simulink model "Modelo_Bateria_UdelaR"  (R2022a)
settings: Solver=VariableStepAuto  StartTime=0.0  StopTime=inf  RelTol=1e-3
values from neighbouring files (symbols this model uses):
  a = x(1)    [Cycling_LiFePO4.m]    (also in Parametros_A123.m = 2.09162011618e-08; Parametros_A123_pack.m = 2.09162011618e-08)
  A = @(x) x(1)    [Cycling_LiFePO4.m]    (also in LMFsolve.m = J'*J; Parametros_A123.m = 0.3446; Parametros_A123_pack.m = 0.3446)
  Alpha = 1093.6    [Parametros_A123.m]    (also in Parametros_A123_pack.m)
  b = x(2)    [Cycling_LiFePO4.m]    (also in Parametros_A123.m = -1.21794950859e-05; Parametros_A123_pack.m = -1.21794950859e-05)
  B = @(x) x(2)    [Cycling_LiFePO4.m]    (also in Parametros_A123.m = 13.0435; Parametros_A123_pack.m = 13.0435)
  Beta = 8390.6    [Parametros_A123.m]    (also in Parametros_A123_pack.m)
  c = x(3)    [Cycling_LiFePO4.m]    (also in Parametros_A123.m = 0.00180276688394; Parametros_A123_pack.m = 0.00180276688394)
  d = x(4)    [Cycling_LiFePO4.m]    (also in LMFsolve.m = (A+l*D)\v; Parametros_A123.m = -1.70817769928e-06; Parametros_A123_pack.m = -1.70817769928e-06)
  dE_dT = 0.000010001    (= 1.0001e-05)    [Parametros_A123.m]    (also in Parametros_A123_pack.m)
  dQ_dT = 0.0037    [Parametros_A123.m]    (also in Parametros_A123_pack.m)
  Eo = 3.3678    [Parametros_A123.m]    (also in Parametros_A123_pack.m)
  f = x(1)*Q0    [Calendar_LiFePO4.m]    (also in Cycling_LiFePO4.m = f*(exp(g)-1)/(g*exp(0.5)); LMFsolve.m = '; Parametros_A123.m = 5980801.16971; Parametros_A123_pack.m = 5980801.16971)
  g = x(2)    [Calendar_LiFePO4.m]    (also in Cycling_LiFePO4.m = 0.689770643187; Parametros_A123.m = 0.689770643187; Parametros_A123_pack.m = 0.689770643187)
  h = x(3)    [Calendar_LiFePO4.m]    (also in Cycling_LiFePO4.m = -6464.71191685; Parametros_A123.m = -6464.71191685; Parametros_A123_pack.m = -6464.71191685)
  Ic = Q*5/Q    (= 5)    [Parametros_A123.m]    (also in Parametros_A123_pack.m = 69)
  Id = Q*3/Q    (= 3)    [Parametros_A123.m]    (also in Parametros_A123_pack.m = 69)
  K = 0.0029    [Parametros_A123.m]    (also in Parametros_A123_pack.m)
  Kc = 0.1    [Parametros_A123.m]    (also in Parametros_A123_pack.m)
  Np = 1    [Parametros_A123.m]    (also in Parametros_A123_pack.m = 10)
  Ns = 1    [Parametros_A123.m]    (also in Parametros_A123_pack.m = 200)
  Q = zeros(9,12)    [Calendar_LiFePO4.m]    (also in Cycling_LiFePO4.m = transpose(Q); Parametros_A123.m = 2.3; Parametros_A123_pack.m = 2.3)
  Rohm = 0.01    [Parametros_A123.m]    (also in Parametros_A123_pack.m)
  Rout = 0.6    [Parametros_A123.m]    (also in Parametros_A123_pack.m)
  SOC0 = 100    [Parametros_A123.m]    (also in Parametros_A123_pack.m)
  Ta = 45    [Parametros_A123.m]    (also in Parametros_A123_pack.m = 25)
  Tcrit = 65    [Parametros_A123.m]    (also in Parametros_A123_pack.m)
  Tf = 10    [Parametros_A123.m]    (also in Parametros_A123_pack.m)
  To = 298.15    [Parametros_A123.m]    (also in Parametros_A123_pack.m)
  Tth = 1000    [Parametros_A123.m]    (also in Parametros_A123_pack.m)
  Umin = 2    [Parametros_A123.m]    (also in Parametros_A123_pack.m = 400)
  w = 1.5    [Parametros_A123.m]    (also in Parametros_A123_pack.m)
undefined symbols (not defined in the file or in its folder): nthroot
libraries: simulink x3, spsControlledCurrentSourceLib x3, spsControlledVoltageSourceLib x2, spsCurrentMeasurementLib x2, dspswit3 x1, simulink_extras x1, spsVoltageMeasurementLib x1, spspowerguiLib x1

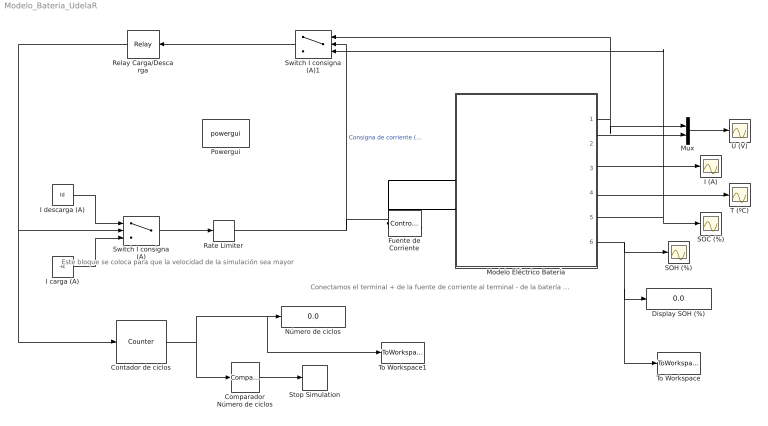
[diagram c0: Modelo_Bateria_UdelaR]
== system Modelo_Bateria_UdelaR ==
  note: Este bloque se coloca para que la velocidad de la simulación sea mayor
  note: Conectamos el terminal + de la fuente de corriente al terminal - de la batería y viceversa porque consideramos i > 0 durante la descarga.
  Comparador Número de ciclos : simulink/Logic and Bit Operations/Compare To Constant  relop=>=  const=1000  OutDataTypeStr=boolean
  Contador de ciclos : dspswit3/Counter  Direction=Up  CountEvent=Either edge  CounterSize=User defined  MaxCount=10000  InitialCount=0  Output=Count  HitValue=32  ResetInput=off  SamplesPerFrame=1  Ts=1  CntDtype=double  HitDtype=Logical
  Display SOH (%) : Display
  Fuente de Corriente : spsControlledCurrentSourceLib/Controlled Current Source  Initialize=on  Source_Type=AC  Amplitude=0  Phase=0  Frequency=0  Measurements=None
  I (A) : Scope
  I carga (A) : Constant  Value=-Ic
  I descarga (A) : Constant  Value=Id
  Modelo Eléctrico Batería : Subsystem  VariantControl=Continuous
  Mux : Mux  Inputs=2
  Número de ciclos : Display
  Powergui : spspowerguiLib/powergui  Priority=1  SimulationMode=Continuous  SampleTime=50e-6  frequency=60  Iterations=50  frequencyindice=0  Pbase=100e6  ErrMax=1e-4  UnitsV=kV  UnitsW=MW  buscounter=0  FunctionMessages=off  echomessages=off  EnableUseOfTLC=off  CurrentSourceSwitches=off  DisableSnubberDevices=off  DisableRonSwitches=off  DisableVfSwitches=off  DisplayEquations=off  AutomaticDiscreteSolvers=off  SolverType=Tustin/Backward Euler (TBE)  Interpol=off  ExternalGateDelay=off  methode=off  Ts=100  x0status=blocks  SPID=on  SwTol=0  HookPort=off  NonlinearTolerance=0  nMaxIteration=15  ContinueOnMaxIteration=off  RestoreLinks=warning  ResistiveCurrentMeasurement=off  Frange=[0:2:500]  Ylog=off  Xlog=on  ShowGrid=off  save=off  variable=ZData  structure=0  ZoomFFT=off  StartTime=0.0  cycles=1  DisplayStyle=1  fundamental=60  FreqAxis=off  MaxFrequency=1000  frequencyindicesteady=1  RmsSteady=1  display=off
  Rate Limiter : RateLimiter  RisingSlewLimit=inf  FallingSlewLimit=-inf  SampleTimeMode=inherited
  Relay Carga/Descarga : Relay  OnSwitchValue=100  OffSwitchValue=Umin
  SOC (%) : Scope
  SOH (%) : Scope
  Stop Simulation : Stop
  Switch I consigna (A) : Switch  Criteria=u2 > Threshold  Threshold=0.5
  Switch I consigna (A)1 : Switch  Criteria=u2 > Threshold
  T (ºC) : Scope
  To Workspace : ToWorkspace  VariableName=SOH  SampleTime=7000
  To Workspace1 : ToWorkspace  VariableName=Nciclos  SampleTime=7000
  U (V) : Scope
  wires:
  Rate Limiter/1 -> Switch I consigna (A)1/2, Fuente de Corriente/1  "Consigna de corriente (A)"
  Switch I consigna (A)/1 -> Rate Limiter/1
  Relay Carga/Descarga/1 -> Contador de ciclos/1, Switch I consigna (A)/2
  I carga (A)/1 -> Switch I consigna (A)/3
  I descarga (A)/1 -> Switch I consigna (A)/1
  Modelo Eléctrico Batería/5(SOC) -> Switch I consigna (A)1/3, SOC (%)/1
  Modelo Eléctrico Batería/6(SOH) -> SOH (%)/1, To Workspace/1, Display SOH (%)/1
  Comparador Número de ciclos/1 -> Stop Simulation/1
  Contador de ciclos/1 -> To Workspace1/1, Número de ciclos/1, Comparador Número de ciclos/1
  Modelo Eléctrico Batería/2(E) -> Mux/2
  Modelo Eléctrico Batería/3(I medida) -> I (A)/1
  Modelo Eléctrico Batería/4(T) -> T (ºC)/1
  Switch I consigna (A)1/1 -> Relay Carga/Descarga/1
  Modelo Eléctrico Batería/1(U) -> Switch I consigna (A)1/1, Mux/1
  Mux/1 -> U (V)/1
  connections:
  Fuente de Corriente/RConn1 -- Modelo Eléctrico Batería/LConn2
  Modelo Eléctrico Batería/LConn1 -- Fuente de Corriente/LConn1

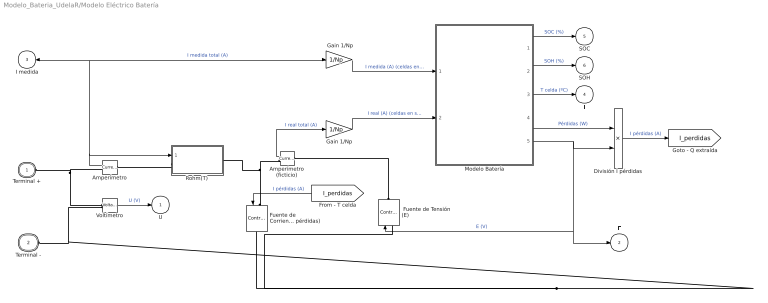
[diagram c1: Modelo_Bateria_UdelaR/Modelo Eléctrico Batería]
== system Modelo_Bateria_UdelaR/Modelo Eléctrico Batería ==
  "  Gain 1/Np " : Gain  Gain=1/Np
  " Fuente de Tensión (E)" : spsControlledVoltageSourceLib/Controlled Voltage Source  Initialize=on  Source_Type=AC  Amplitude=0  Phase=0  Frequency=0  Measurements=None
  " Gain 1/Np " : Gain  Gain=1/Np
  Amperímetro : spsCurrentMeasurementLib/Current Measurement  PhasorSimulation=off  OutputType=Complex  PSBequivalent=0
      link override do not delete this gain: Gain=1
  Amperímetro (ficticio) : spsCurrentMeasurementLib/Current Measurement  PhasorSimulation=off  OutputType=Complex  PSBequivalent=0
  División I pérdidas : Product  Inputs=*/
  Fuente de Corriente (de pérdidas) : spsControlledCurrentSourceLib/Controlled Current Source  Initialize=on  Source_Type=AC  Amplitude=0  Phase=0  Frequency=0  Measurements=None
  Modelo Batería : Subsystem  VariantControl=Continuous
  Rohm(T) : Subsystem  VariantControl=Continuous
  Voltímetro : spsVoltageMeasurementLib/Voltage Measurement  PhasorSimulation=off  OutputType=Complex  PSBequivalent=0
  Terminal + : PMIOPort  Side=Left
  Terminal - : PMIOPort  Port=2  Side=Left
  U : Outport  VectorParamsAs1DForOutWhenUnconnected=off
  E : Outport  Port=2  VectorParamsAs1DForOutWhenUnconnected=off
  I medida : Outport  Port=3  VectorParamsAs1DForOutWhenUnconnected=off
  T : Outport  Port=4  VectorParamsAs1DForOutWhenUnconnected=off
  SOC : Outport  Port=5  VectorParamsAs1DForOutWhenUnconnected=off
  SOH : Outport  Port=6  VectorParamsAs1DForOutWhenUnconnected=off
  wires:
  Voltímetro/1 -> U/1  "U (V)"
  Amperímetro/1 -> "  Gain 1/Np "/1, I medida/1, Rohm(T)/1(I medida)  "I medida total (A)"
  Amperímetro (ficticio)/1 -> " Gain 1/Np "/1  "I real total (A)"
  [I_perdidas] -> Fuente de Corriente (de pérdidas)/1  "I pérdidas (A)"
  Modelo Batería/1(SOC) -> SOC/1  "SOC (%)"
  Modelo Batería/2(SOH) -> SOH/1  "SOH (%)"
  Modelo Batería/3(T) -> T/1  "T celda (ºC)"
  Modelo Batería/5(E) -> División I pérdidas/2, " Fuente de Tensión (E)"/1, E/1  "E (V)"
  Modelo Batería/4(P Temp) -> División I pérdidas/1  "Pérdidas (W)"
  División I pérdidas/1 -> [I_perdidas]  "I pérdidas (A)"
  " Gain 1/Np "/1 -> Modelo Batería/2(I real)  "I real (A) (celdas en serie)"
  "  Gain 1/Np "/1 -> Modelo Batería/1(I medida)  "I medida (A) (celdas en serie)"
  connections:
  Voltímetro/LConn1 -- Terminal +/RConn1 -- Amperímetro/RConn1
  Voltímetro/LConn2 -- " Fuente de Tensión (E)"/LConn1 -- Fuente de Corriente (de pérdidas)/RConn1 -- Terminal -/RConn1
  Rohm(T)/LConn1 -- Amperímetro/LConn1
  Fuente de Corriente (de pérdidas)/LConn1 -- Amperímetro (ficticio)/RConn1 -- Rohm(T)/RConn1
  " Fuente de Tensión (E)"/RConn1 -- Amperímetro (ficticio)/LConn1

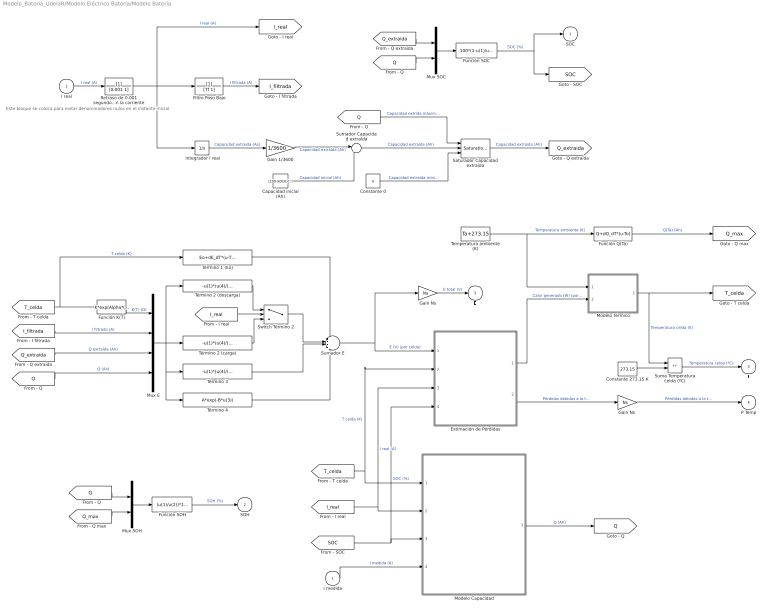
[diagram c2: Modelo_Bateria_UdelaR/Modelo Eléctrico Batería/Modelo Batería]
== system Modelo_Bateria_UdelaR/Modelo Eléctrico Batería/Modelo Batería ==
  note: Este bloque se coloca para evitar denominadores nulos en el instante inicial
  I medida : Inport
  I real : Inport  Port=2
  " Gain Ns  " : Gain  Gain=Ns
  " Integrador I real" : Integrator
  Capacidad inicial (Ah) : Constant  Value=(100-SOC0)*Q/100
  Constante 0 : Constant  Value=0
  Constante 273.15 K : Constant  Value=273.15
  Estimación de Pérdidas : Subsystem
  Filtro Paso Bajo : TransferFcn  Denominator=[Tf 1]
  Función K(T) : Fcn  Expr=K*exp(Alpha*((1/u)-(1/To)))
  Función Q(Ta) : Fcn  Expr=Q+dQ_dT*(u-To)
  Función SOC : Fcn  Expr=100*(1-u(1)/u(2))
  Función SOH : Fcn  Expr=(u(1)/u(2))*100
  Gain 1/3600 : Gain  Gain=1/3600
  Gain Ns : Gain  Gain=Ns
  Modelo Capacidad : Subsystem  VariantControl=Continuous
  Modelo Térmico : Subsystem  VariantControl=Continuous
  Mux E : Mux
  Mux SOC : Mux  Inputs=2
  Mux SOH : Mux  Inputs=2
  Retraso de 0.001 segundos en la corriente : TransferFcn  Denominator=[0.001 1]
  Saturador Capacidad extraída : simulink/Discontinuities/Saturation Dynamic  OutMin=[]  OutMax=[]  OutDataTypeStr=Inherit: Same as second input  OutDataType=fixdt(1, 16)  OutScaling=2^-10  DoSatur=off
  Suma Temperatura celda (ºC) : Sum  Inputs=+-
  Sumador Capacidad extraída : Sum  Inputs=|++
  Sumador E : Sum  Inputs=++++
  Switch Término 2 : Switch  Criteria=u2 > Threshold
  Temperatura ambiente (K) : Constant  Value=Ta+273.15
  Término 1 (Eo) : Fcn  Expr=Eo+dE_dT*(u-To)
  Término 2 (carga) : Fcn  Expr=-u(1)*(u(4)/(u(3)+Kc*u(4)))*u(2)
  Término 2 (descarga) : Fcn  Expr=-u(1)*(u(4)/(u(4)-u(3)))*u(2)
  Término 3 : Fcn  Expr=-u(1)*(u(4)/(u(4)-u(3)))*u(3)
  Término 4 : Fcn  Expr=A*exp(-B*u(3))
  SOC : Outport  VectorParamsAs1DForOutWhenUnconnected=off
  SOH : Outport  Port=2  VectorParamsAs1DForOutWhenUnconnected=off
  T : Outport  Port=3  VectorParamsAs1DForOutWhenUnconnected=off
  P Temp : Outport  Port=4  VectorParamsAs1DForOutWhenUnconnected=off
  E : Outport  Port=5  VectorParamsAs1DForOutWhenUnconnected=off
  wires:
  Filtro Paso Bajo/1 -> [I_filtrada]  "I filtrada (A)"
  " Integrador I real"/1 -> Gain 1/3600/1  "Capacidad extraída (As)"
  [Q] -> Saturador Capacidad extraída/1  "Capacidad extrída máxima (Ah)"
  Constante 0/1 -> Saturador Capacidad extraída/3  "Capacidad extraída mínima (Ah)"
  Saturador Capacidad extraída/1 -> [Q_extraida]  "Capacidad extraída (Ah)"
  [T_celda] -> Término 1 (Eo)/1, Función K(T)/1  "T celda (K)"
  Función K(T)/1 -> Mux E/1  "K(T) (Ω)"
  [I_filtrada] -> Mux E/2  "I filtrada (A)"
  [Q_extraida] -> Mux E/3  "Q extraída (Ah)"
  [Q] -> Mux E/4  "Q (Ah)"
  Término 2 (descarga)/1 -> Switch Término 2/1
  Término 2 (carga)/1 -> Switch Término 2/3
  [I_real] -> Switch Término 2/2
  Término 4/1 -> Sumador E/4
  Switch Término 2/1 -> Sumador E/2
  Mux E/1 -> Término 4/1, Término 3/1, Término 2 (descarga)/1, Término 2 (carga)/1
  Término 1 (Eo)/1 -> Sumador E/1
  Sumador E/1 -> Gain Ns/1, Estimación de Pérdidas/1(E)  "E (V) (por celda)"
  Estimación de Pérdidas/2(P Temp) -> " Gain Ns  "/1  "Pérdidas debidas a la temperatura (W) (por celda)"
  " Gain Ns  "/1 -> P Temp/1  "Pérdidas debidas a la temperatura (W) (celdas en serie)"
  Estimación de Pérdidas/1(H) -> Modelo Térmico/2(H)  "Calor generado (W) (por celda)"
  Temperatura ambiente (K)/1 -> Función Q(Ta)/1, Modelo Térmico/1(Ta)  "Temperatura ambiente (K)"
  Función Q(Ta)/1 -> [Q_max]  "Q(Ta) (Ah)"
  Modelo Térmico/1(T) -> [T_celda], Suma Temperatura celda (ºC)/1  "Temperatura celda (K)"
  Suma Temperatura celda (ºC)/1 -> T/1  "Temperatura celda (ºC)"
  Constante 273.15 K/1 -> Suma Temperatura celda (ºC)/2
  [Q_extraida] -> Mux SOC/1
  [Q] -> Mux SOC/2
  [Q] -> Mux SOH/1
  [Q_max] -> Mux SOH/2
  Mux SOH/1 -> Función SOH/1
  Mux SOC/1 -> Función SOC/1
  Función SOH/1 -> SOH/1  "SOH (%)"
  Función SOC/1 -> SOC/1, [SOC]  "SOC (%)"
  Modelo Capacidad/1(Q) -> [Q]  "Q (Ah)"
  Gain Ns/1 -> E/1  "E total (V)"
  Retraso de 0.001 segundos en la corriente/1 -> " Integrador I real"/1, [I_real], Filtro Paso Bajo/1  "I real (A)"
  Gain 1/3600/1 -> Sumador Capacidad extraída/1  "Capacidad extraída (Ah)"
  Capacidad inicial (Ah)/1 -> Sumador Capacidad extraída/2  "Capacidad inicial (Ah)"
  Sumador Capacidad extraída/1 -> Saturador Capacidad extraída/2  "Capacidad extraída (Ah)"
  Término 3/1 -> Sumador E/3
  [T_celda] -> Estimación de Pérdidas/2(T), Modelo Capacidad/1(T)  "T celda (K)"
  [I_real] -> Estimación de Pérdidas/3(I real), Modelo Capacidad/2(I real)  "I real (A)"
  [SOC] -> Estimación de Pérdidas/4(SOC), Modelo Capacidad/3(SOC)  "SOC (%)"
  I real/1 -> Retraso de 0.001 segundos en la corriente/1  "I real (A)"
  I medida/1 -> Modelo Capacidad/4(I medida)  "I medida (A)"

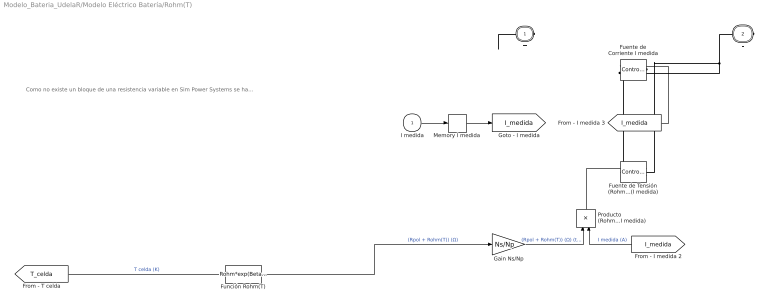
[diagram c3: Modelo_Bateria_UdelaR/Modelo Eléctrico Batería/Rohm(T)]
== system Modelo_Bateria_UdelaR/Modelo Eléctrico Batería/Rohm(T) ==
  note: Como no existe un bloque de una resistencia variable en Sim Power Systems se ha recreado una. Para ello se se coloca en bornes del bloque una tensión igual a la resistencia deseada y se multiplica por la corriente que circula por ella. Por lo tanto, el cociente de U/I obtenido es igual a R. Nótese que la polarización de los términales es la inversa, esto se debe a que se ha considerado que la corriente durante la descarga es i > 0.
  I medida : Inport
  Fuente de Corriente I medida : spsControlledCurrentSourceLib/Controlled Current Source  Initialize=on  Source_Type=AC  Amplitude=0  Phase=0  Frequency=0  Measurements=None
  Fuente de Tensión (Rohm+Rpol)*(I medida) : spsControlledVoltageSourceLib/Controlled Voltage Source  Initialize=on  Source_Type=AC  Amplitude=0  Phase=0  Frequency=0  Measurements=None
  Función Rohm(T) : Fcn  Expr=Rohm*exp(Beta*((1/u)-(1/To)))
  Gain Ns/Np : Gain  Gain=Ns/Np
  Memory I medida : Memory
  "Producto (Rohm+Rpol)*(I medida) " : Product
  + : PMIOPort  Side=Left
  - : PMIOPort  Port=2  Side=Right
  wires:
  [T_celda] -> Función Rohm(T)/1  "T celda (K)"
  "Producto (Rohm+Rpol)*(I medida) "/1 -> Fuente de Tensión (Rohm+Rpol)*(I medida)/1
  Función Rohm(T)/1 -> Gain Ns/Np/1  "(Rpol + Rohm(T)) (Ω)"
  [I_medida] -> "Producto (Rohm+Rpol)*(I medida) "/2  "I medida (A)"
  [I_medida] -> Fuente de Corriente I medida/1
  Gain Ns/Np/1 -> "Producto (Rohm+Rpol)*(I medida) "/1  "(Rpol + Rohm(T)) (Ω) (total de la batería)"
  I medida/1 -> Memory I medida/1
  Memory I medida/1 -> [I_medida]
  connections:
  -/RConn1 -- Fuente de Tensión (Rohm+Rpol)*(I medida)/RConn1 -- Fuente de Corriente I medida/LConn1
  Fuente de Corriente I medida/RConn1 -- Fuente de Tensión (Rohm+Rpol)*(I medida)/LConn1 -- +/RConn1

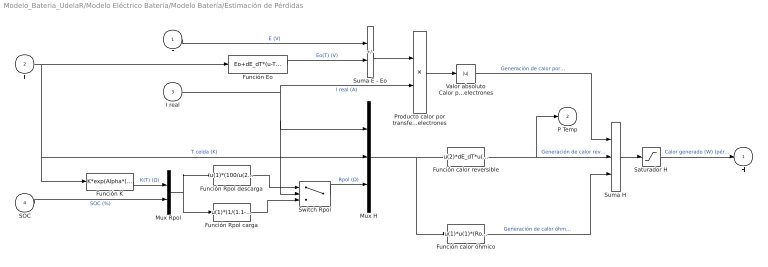
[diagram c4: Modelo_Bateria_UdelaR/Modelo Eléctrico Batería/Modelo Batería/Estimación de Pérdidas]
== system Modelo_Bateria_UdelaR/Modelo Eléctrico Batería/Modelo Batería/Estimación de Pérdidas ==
  E : Inport
  T : Inport  Port=2
  I real : Inport  Port=3
  SOC : Inport  Port=4
  Función Eo : Fcn  Expr=Eo+dE_dT*(u-To)
  Función K : Fcn  Expr=K*exp(Alpha*((1/u)-(1/To)))
  Función Rpol carga : Fcn  Expr=u(1)*(1/(1.1-(u(2)/100)))
  Función Rpol descarga : Fcn  Expr=u(1)*(100/u(2))
  Función calor reversible : Fcn  Expr=u(2)*dE_dT*u(1)
  Función calor óhmico : Fcn  Expr=u(1)*u(1)*(Rohm*exp(Beta*((1/u(2))-(1/To)))+u(3))
  Mux H : Mux  Inputs=3
  Mux Rpol : Mux  Inputs=2
  Producto calor por transferencia de electrones : Product
  Saturador H : Saturate  UpperLimit=inf  LowerLimit=0
  Suma E - Eo : Sum  Inputs=-+
  Suma H : Sum  Inputs=+++
  Switch Rpol : Switch  Criteria=u2 > Threshold
  Valor absoluto Calor por transferencia de electrones : Abs
  H : Outport  VectorParamsAs1DForOutWhenUnconnected=off
  P Temp : Outport  Port=2  VectorParamsAs1DForOutWhenUnconnected=off
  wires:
  Función calor óhmico/1 -> Suma H/3  "Generación de calor óhmica (W) (pérdidas)"
  Función calor reversible/1 -> Suma H/2, P Temp/1  "Generación de calor reversible (W) (pérdidas)"
  Valor absoluto Calor por transferencia de electrones/1 -> Suma H/1  "Generación de calor por transferencia de electrones (W) (pérdidas)"
  Saturador H/1 -> H/1  "Calor generado (W) (pérdidas)"
  Función Rpol descarga/1 -> Switch Rpol/1
  Mux H/1 -> Función calor óhmico/1, Función calor reversible/1
  I real/1 -> Producto calor por transferencia de electrones/2, Switch Rpol/2, Mux H/1  "I real (A)"
  T/1 -> Función Eo/1, Función K/1, Mux H/2  "T celda (K)"
  Función Eo/1 -> Suma E - Eo/2  "Eo(T) (V)"
  E/1 -> Suma E - Eo/1  "E (V)"
  Suma E - Eo/1 -> Producto calor por transferencia de electrones/1
  Producto calor por transferencia de electrones/1 -> Valor absoluto Calor por transferencia de electrones/1
  Switch Rpol/1 -> Mux H/3  "Rpol (Ω)"
  Mux Rpol/1 -> Función Rpol carga/1, Función Rpol descarga/1
  Función K/1 -> Mux Rpol/1  "K(T) (Ω)"
  SOC/1 -> Mux Rpol/2  "SOC (%)"
  Suma H/1 -> Saturador H/1
  Función Rpol carga/1 -> Switch Rpol/3

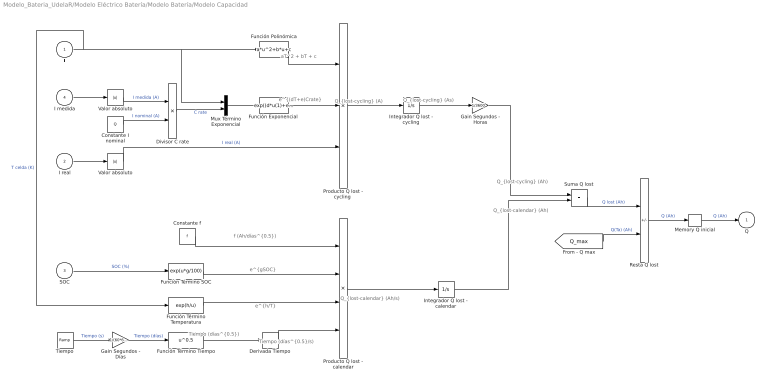
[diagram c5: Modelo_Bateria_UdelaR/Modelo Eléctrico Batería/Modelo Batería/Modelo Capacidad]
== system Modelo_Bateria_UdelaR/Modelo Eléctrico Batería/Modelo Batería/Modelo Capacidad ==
  note: aT^2 + bT + c
  note: e^{(dT+e)Crate}
  note: Q_{lost-cycling} (A)
  note: Q_{lost-cycling} (As)
  note: Q_{lost-cycling} (Ah)
  note: Tiempo (días^{0.5})
  note: e^{gSOC}
  note: e^{h/T}
  note: f (Ah/días^{0.5})
  note: Tiempo (días^{0.5}/s)
  note: Q_{lost-calendar} (Ah/s)
  note: Q_{lost-calendar} (Ah)
  T : Inport
  I real : Inport  Port=2
  SOC : Inport  Port=3
  I medida : Inport  Port=4
  " Valor absoluto " : Abs
  Constante I nominal : Constant  Value=Q
  Constante f : Constant  Value=f
  Derivada Tiempo : Derivative
  Divisor C rate : Product  Inputs=*/
  "Función Exponencial " : Fcn  Expr=exp((d*u(1)+e)*u(2))
  Función Polinómica : Fcn  Expr=a*u^2+b*u+c
  Función Término SOC : Fcn  Expr=exp(u*g/100)
  Función Término Temperatura : Fcn  Expr=exp(h/u)
  Función Término Tiempo : Fcn  Expr=u^0.5
  Gain Segundos - Días : Gain  Gain=1/(60*60*24)
  Gain Segundos - Horas : Gain  Gain=1/3600
  Integrador Q lost - calendar : Integrator
  Integrador Q lost - cycling : Integrator
  Memory Q inicial : Memory  InitialCondition=Q
  Mux Término Exponencial : Mux  Inputs=2
  Producto Q lost - calendar : Product  Inputs=4
  "Producto Q lost - cycling " : Product  Inputs=3
  Resta Q lost : Sum  Inputs=-+
  Suma Q lost : Sum
  Tiempo : simulink/Sources/Ramp  slope=12/w  start=0  InitialOutput=0
  Valor absoluto : Abs
  Q : Outport  VectorParamsAs1DForOutWhenUnconnected=off
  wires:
  Memory Q inicial/1 -> Q/1  "Q (Ah)"
  Resta Q lost/1 -> Memory Q inicial/1  "Q (Ah)"
  Constante I nominal/1 -> Divisor C rate/2  "I nominal (A)"
  I real/1 -> " Valor absoluto "/1
  Divisor C rate/1 -> Mux Término Exponencial/2  "C rate"
  [Q_max] -> Resta Q lost/2  "Q(Ta) (Ah)"
  Función Término SOC/1 -> Producto Q lost - calendar/2
  Gain Segundos - Días/1 -> Función Término Tiempo/1  "Tiempo (días)"
  Producto Q lost - calendar/1 -> Integrador Q lost - calendar/1
  SOC/1 -> Función Término SOC/1  "SOC (%)"
  "Producto Q lost - cycling "/1 -> Integrador Q lost - cycling/1
  Integrador Q lost - cycling/1 -> Gain Segundos - Horas/1
  T/1 -> Mux Término Exponencial/1, Función Polinómica/1, Función Término Temperatura/1  "T celda (K)"
  Función Término Tiempo/1 -> Derivada Tiempo/1
  Constante f/1 -> Producto Q lost - calendar/1
  Derivada Tiempo/1 -> Producto Q lost - calendar/4
  " Valor absoluto "/1 -> "Producto Q lost - cycling "/3  "I real (A)"
  I medida/1 -> Valor absoluto/1
  Valor absoluto/1 -> Divisor C rate/1  "I medida (A)"
  Mux Término Exponencial/1 -> "Función Exponencial "/1
  Función Polinómica/1 -> "Producto Q lost - cycling "/1
  "Función Exponencial "/1 -> "Producto Q lost - cycling "/2
  Gain Segundos - Horas/1 -> Suma Q lost/1
  Función Término Temperatura/1 -> Producto Q lost - calendar/3
  Tiempo/1 -> Gain Segundos - Días/1  "Tiempo (s)"
  Integrador Q lost - calendar/1 -> Suma Q lost/2
  Suma Q lost/1 -> Resta Q lost/1  "Q lost (Ah)"

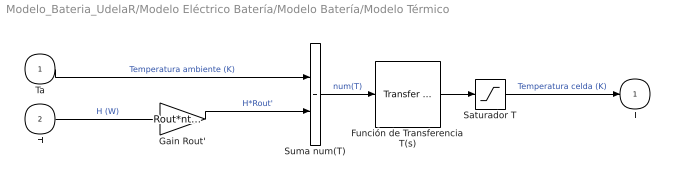
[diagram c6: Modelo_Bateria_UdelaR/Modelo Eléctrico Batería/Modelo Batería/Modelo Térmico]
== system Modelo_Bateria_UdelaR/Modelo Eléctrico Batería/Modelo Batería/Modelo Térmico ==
  Ta : Inport
  H : Inport  Port=2
  Función de Transferencia T(s) : simulink_extras/Additional Linear/Transfer Fcn (with initial outputs)  N=[1]  D="[Tth  1]"  Y0=Ta+273.15  U0=0
  Gain Rout' : Gain  Gain=Rout*nthroot(0.5*Ns, 6)
  Saturador T : Saturate  UpperLimit=Tcrit+273.15  LowerLimit=0
  Suma num(T) : Sum
  T : Outport  VectorParamsAs1DForOutWhenUnconnected=off
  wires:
  Suma num(T)/1 -> Función de Transferencia T(s)/1  "num(T)"
  Función de Transferencia T(s)/1 -> Saturador T/1
  Gain Rout'/1 -> Suma num(T)/2  "H*Rout'"
  H/1 -> Gain Rout'/1  "H (W)"
  Saturador T/1 -> T/1  "Temperatura celda (K)"
  Ta/1 -> Suma num(T)/1  "Temperatura ambiente (K)"
